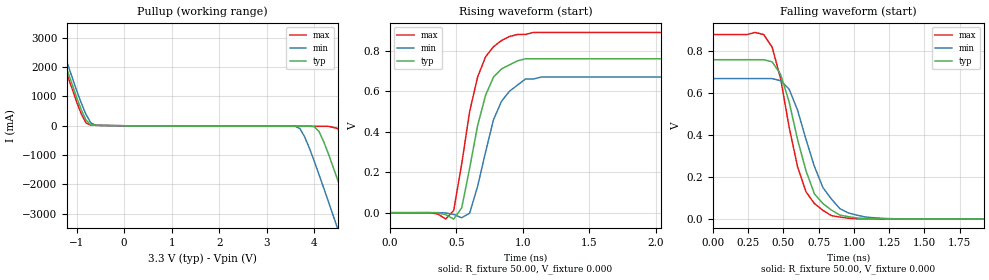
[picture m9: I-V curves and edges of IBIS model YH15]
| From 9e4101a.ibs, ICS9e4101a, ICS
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|   Model YH15
[Model]   YH15
Model_type   Open_source
Polarity   Inverting
C_comp   5.50pF   5.00pF   6.00pF
[Temperature Range]   27.00   70.00   0.000
[Voltage Range]   3.30V   3.00V   3.70V
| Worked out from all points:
|   slope of the pullup table from 0 to 0.495 V, typ, clamps not added: 56.2 ohm
|   rising waveform, R_fixture 50.00, V_fixture 0.000: 20-80 % time 159ps typ, 169ps min, 161ps max; typ from 0 V to 0.76 V
|   falling waveform, R_fixture 50.00, V_fixture 0.000: 20-80 % time 185ps typ, 207ps min, 171ps max; typ from 0.76 V to 0 V
[Pullup]
| voltage   I(typ)   I(min)   I(max)
-3.3V     12.3A      12.52A     12.16A
-1.7V     4.31A      4.55A      4.16A
-1.5V     3.33A      3.58A      3.17A
-900mV    540mA      770mA      400mA
-700mV    28.62mA    98.17mA    20.44mA
3.7V      -15.27mA   -98.55mA   -17.78mA
4.1V      -190mA     -1.66A     -17.81mA
4.5V      -1.87A     -3.54A     -94.69mA
4.7V      -2.82A     -4.51A     -810mA
4.9V      -3.78A     -5.48A     -1.72A
5.3V      -5.73A     -7.43A     -3.63A
6.6V      -12.13A    -13.84A    -10.01A
[Ramp]
| variable   typ   min   max
dV/dt_r   0.46/0.15n   0.40/0.17n   0.53/0.15n
dV/dt_f   0.45/0.17n   0.40/0.20n   0.53/0.16n
R_load = 50.00
[Rising Waveform]
R_fixture = 50.00
V_fixture = 0.000
V_fixture_min = 0.000
V_fixture_max = 0.000
| time   V(typ)   V(min)   V(max)
0s        0V         0V         0V
420ps     -9.86mV    -1.08mV    -31.06mV
480ps     -31.44mV   -8.74mV    11.06mV
540ps     23.78mV    -24.96mV   240mV
600ps     220mV      -2.43mV    500mV
660ps     430mV      130mV      670mV
780ps     670mV      460mV      820mV
900ps     730mV      600mV      870mV
1.14ns    760mV      670mV      890mV
3ns       760mV      670mV      890mV
[Falling Waveform]
R_fixture = 50.00
V_fixture = 0.000
V_fixture_min = 0.000
V_fixture_max = 0.000
| time   V(typ)   V(min)   V(max)
0s        760mV      670mV      880mV
300ps     760mV      670mV      890mV
420ps     750mV      670mV      820mV
480ps     690mV      660mV      670mV
540ps     560mV      620mV      440mV
660ps     230mV      380mV      130mV
720ps     120mV      250mV      73.59mV
840ps     43.05mV    95.69mV    16.34mV
1.14ns    1.56mV     6.17mV     630uV
3ns       3.97uV     -14.51uV   1.38uV
